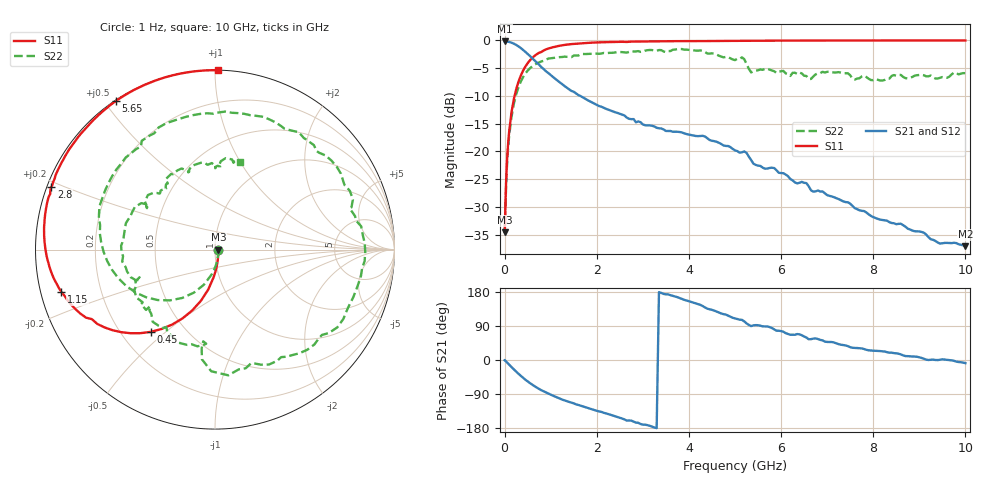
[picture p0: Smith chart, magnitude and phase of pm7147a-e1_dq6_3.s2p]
# GHz S DB R 50
! S-Parameters data
! Freq  dbS11  angS11  dbS21  angS21  dbS12  angS12  dbS22  angS22
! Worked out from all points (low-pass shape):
!   279 points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, 1 Hz to 10 GHz, reference 50 ohm
!   highest |S21| = -0.16 dB at 31.62 kHz (marker M1); lowest = -37.1 dB at 10 GHz (marker M2)
!   |S21| within 3 dB of the highest: start of sweep to 595.1 MHz
!   lowest |S11| = -34.6 dB at 31.62 kHz (marker M3), VSWR 1.04, Z = 51.9 - j0.00469 ohm
!   |S11| at or under -10 dB: start of sweep to 217 MHz
!   |S22| runs from -34.6 to -1.5 dB; largest |S21 - S12| = 1.7e-12
!   S11 on the Smith chart (normalised r, x): 1 Hz: 1.04, -0.00; 450 MHz: 0.32, -0.45; 1.15 GHz: 0.06, -0.13; 2.8 GHz: 0.01, +0.19; 5.65 GHz: 0.00, +0.53; 10 GHz: 0.00, +1.02
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1e-09  -34.61 -0.0  -0.16 0.0  -0.16 0.0  -34.61 -0.0
3.16228e-05  -34.62 -0.1  -0.16 -0.0  -0.16 -0.0  -34.62 -0.1
0.03162278  -25.70 -71.6  -0.18 -4.0  -0.18 -4.0  -26.37 -71.7
0.06309573  -20.17 -84.9  -0.21 -7.9  -0.21 -7.9  -20.93 -87.5
0.15  -12.94 -99.6  -0.40 -18.7  -0.40 -18.7  -13.75 -107.6
0.45  -4.72 -127.9  -2.05 -51.8  -2.05 -51.8  -5.97 -151.7
0.75  -2.21 -147.7  -4.40 -76.5  -4.40 -76.5  -3.95 176.5
1.15  -1.03 -164.6  -7.25 -99.4  -7.25 -99.4  -3.05 144.5
1.7  -0.49 179.7  -10.27 -122.7  -10.27 -122.7  -2.44 111.0
2.15  -0.32 170.2  -12.15 -139.3  -12.15 -139.3  -2.26 85.7
2.8  -0.21 159.0  -14.18 -162.6  -14.18 -162.6  -2.00 51.4
3.35  -0.15 150.9  -15.84 179.0  -15.84 179.0  -1.73 23.6
4.1  -0.11 141.0  -17.17 151.3  -17.17 151.3  -1.78 -19.2
4.55  -0.10 135.6  -18.16 130.3  -18.16 130.3  -2.40 -47.4
5.05  -0.07 130.1  -19.95 108.2  -19.95 108.2  -3.31 -75.5
5.25  -0.07 127.9  -20.27 96.7  -20.27 96.7  -4.22 -96.8
5.65  -0.04 123.7  -23.14 88.6  -23.14 88.6  -5.14 -106.3
6.7  -0.02 113.7  -27.27 56.5  -27.27 56.5  -6.50 -158.9
7.05  -0.01 110.6  -28.03 47.4  -28.03 47.4  -5.62 177.6
7.5  -0.01 106.8  -29.44 33.9  -29.44 33.9  -6.27 147.8
8.35  -0.00 100.2  -32.77 19.2  -32.77 19.2  -6.88 125.4
10  -0.00 89.1  -37.10 -8.3  -37.10 -8.3  -5.91 74.2
